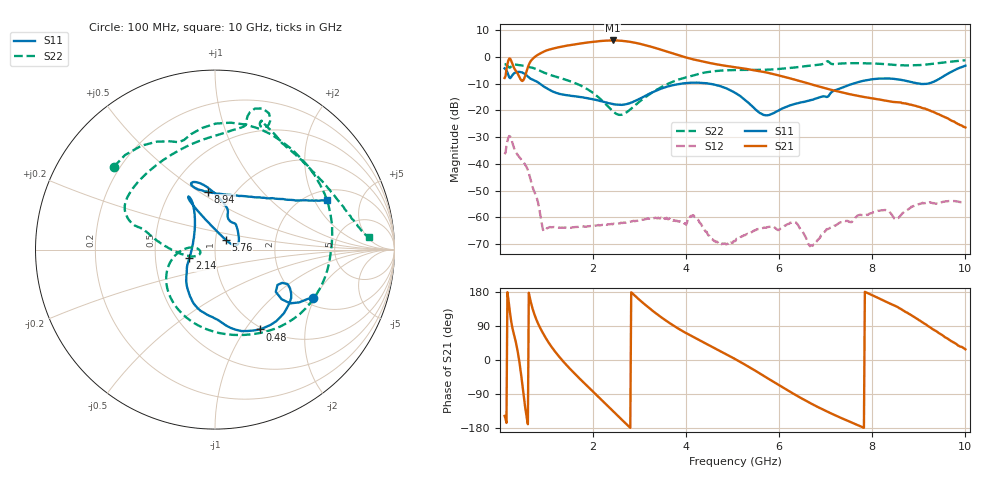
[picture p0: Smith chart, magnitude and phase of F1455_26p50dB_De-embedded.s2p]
! Integrated Device Technology
! Corporate Headquarters
! 6024 Silver Creek Valley Road
! San Jose, CA 95138  USA
! Phone:  1-408-284-8200
! Toll Free:  1-800-223-1366
! Webpage:  http://www.idt.com/
! Timing and RF Division
! 515 Groton Road, Suite 102
! Westford, MA 01886-6024
! Device:  F1455
! Description: 6-bit 0.5 dB Transmit Variable Gain Amplifier
! Frequency:  1400.0 -  2300.00 MHz
! Package:  6x6 mm Thin QFN Plastic Package: 28 pin
! State:  53
! Atten State:  26.5 dB
! Voltage:  +5.00 Volts
! Current:  217.612 mA
! Data:  The device was measured on a the F1455 evaluation board which has
!  individual transmission lines to the RF pins.  Data was collected
!  using a calibrated network analyzer.  The evaluation board was
!  de-embedded using a TRL calibration technique.
!  The reference plane is the edge of the package pin.
!  Pin  1 = CSb
!  Pin  2 = DATA
!  Pin  3 = CLK
!  Pin  4 = RSET
!  Pin  5 = GND
!  Pin  6 = RFIN  = Port 1
!  Pin  7 = GND
!  Pin  8 = NC
!  Pin  9 = NC
!  Pin 10 = NC
!  Pin 11 = NC
!  Pin 12 = NC
!  Pin 13 = NC
!  Pin 14 = /STBY
!  Pin 15 = GND
!  Pin 16 = RFOUT  = Port 2
!  Pin 17 = GND
!  Pin 18 = NC
!  Pin 19 = NC
!  Pin 20 = NC
!  Pin 21 = GND
!  Pin 22 = NC
!  Pin 23 = GND
!  Pin 24 = NC
!  Pin 25 = NC
!  Pin 26 = NC
!  Pin 27 = GND
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# GHz S dB R 50
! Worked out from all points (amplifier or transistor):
!   496 points, 100 MHz to 10 GHz, reference 50 ohm
!   highest |S21| = 6.1 dB at 2.42 GHz (marker M1)
!   |S21| within 3 dB of that: 1.149 GHz to 3.376 GHz (2.227 GHz wide, 98.4 % of centre)
!   unconditionally stable (mu >= 1): start of sweep to end of sweep
!   at 1.74 GHz: K = 365.47, MAG = 5.5 dB, |S12| = -63.3 dB
!   at 5.06 GHz: K = 1388.04, MAG = -2.0 dB, |S12| = -68.8 dB
!   at 10 GHz: K = 730.13, MAG = -17.7 dB, |S12| = -54.3 dB
!   S11 on the Smith chart (normalised r, x): 100 MHz: 2.27, -1.94; 480 MHz: 0.97, -1.17; 2.14 GHz: 0.75, -0.07; 5.76 GHz: 1.12, +0.12; 8.94 GHz: 0.76, +0.54; 10 GHz: 2.44, +2.55
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0.1  -4.30 -26.1  -7.87 -147.5  -36.39 47.3  -2.75 140.7
0.18  -6.69 -36.7  -1.36 161.1  -30.20 -6.4  -3.70 112.5
0.26  -6.98 -25.4  -2.31 89.1  -31.67 -77.0  -3.33 96.0
0.38  -5.64 -42.6  -6.24 23.4  -36.64 -118.4  -3.00 58.2
0.48  -5.85 -60.7  -9.01 -64.0  -38.83 -150.3  -3.25 31.7
0.66  -8.17 -88.0  -1.62 154.4  -46.05 139.9  -3.93 -10.4
0.8  -9.31 -105.9  0.62 101.5  -53.23 109.4  -4.69 -41.6
0.96  -11.29 -123.6  2.11 63.1  -65.08 128.5  -5.98 -71.1
1.34  -14.02 -142.4  3.87 -1.0  -63.75 113.1  -8.15 -121.6
1.76  -15.07 -151.2  5.08 -54.9  -63.30 82.2  -10.93 -158.3
2.14  -16.42 -161.3  5.89 -100.1  -63.00 67.3  -15.45 178.7
2.42  -17.60 -177.1  6.14 -133.7  -62.57 59.2  -20.25 176.7
2.82  -17.08 146.3  5.56 178.7  -61.55 50.3  -19.37 -161.1
3.4  -12.31 118.6  3.00 118.6  -60.08 29.1  -11.98 178.7
4.08  -9.68 116.1  -0.61 65.7  -59.84 16.3  -7.32 163.7
5.06  -13.49 111.9  -3.89 2.0  -68.78 36.0  -4.89 148.4
5.76  -21.78 41.9  -5.96 -48.9  -63.58 27.4  -4.78 119.1
6.34  -17.56 14.1  -8.53 -91.5  -61.73 -16.0  -3.94 89.6
6.7  -16.07 34.4  -10.31 -115.9  -70.41 -162.6  -3.21 78.6
8.36  -8.08 109.4  -16.59 150.0  -57.71 67.5  -2.82 62.5
8.94  -9.80 97.0  -18.35 110.4  -55.22 82.2  -3.14 38.9
10  -3.29 24.0  -26.37 28.1  -54.25 15.1  -1.28 4.6
